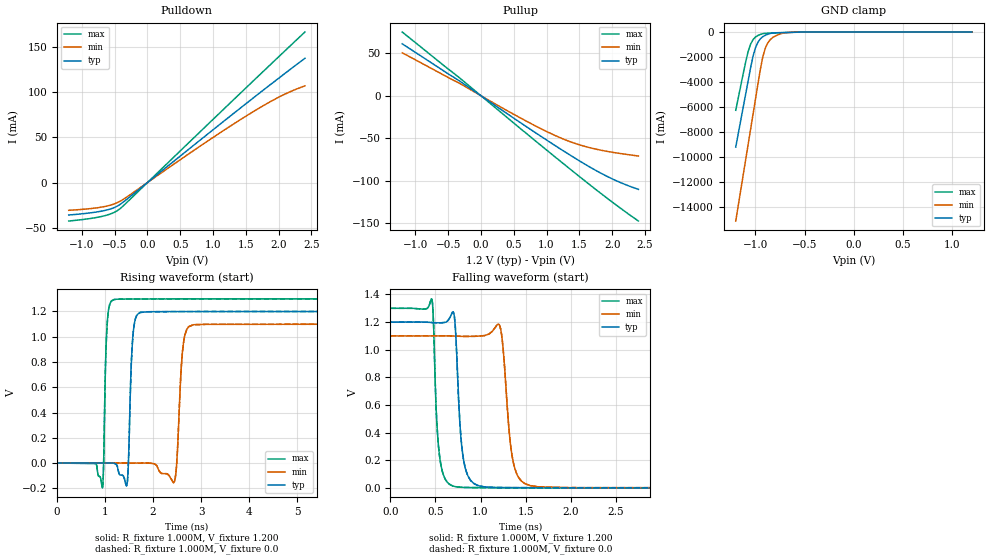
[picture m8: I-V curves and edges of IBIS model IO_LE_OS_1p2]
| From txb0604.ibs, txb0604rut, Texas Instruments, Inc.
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|   Model IO_LE_OS_1p2
[Model] IO_LE_OS_1p2
Model_type 3-state
Polarity   Non-Inverting
Enable   Active-High
Vmeas =  0.600V
Cref =  15.000pF
Rref =  1.000M
Vref =  0.0V
C_comp   3.930pF   3.640pF   4.130pF
[Temperature Range]   27.000   0.125k   -40.000
[Voltage Range]   1.200V   1.100V   1.300V
[Pullup Reference]   1.200V   1.100V   1.300V
[Pulldown Reference]   0.0V   0.0V   0.0V
[POWER Clamp Reference]   1.200V   1.100V   1.300V
[GND Clamp Reference]   0.0V   0.0V   0.0V
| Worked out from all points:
|   slope of the pulldown table from 0 to 0.18 V, typ, clamps not added: 17 ohm
|   slope of the pullup table from 0 to 0.18 V, typ, clamps not added: 18.8 ohm
|   GND clamp passes 1 mA (typ) near -0.43 V on its own axis
|   rising waveform, R_fixture 1.000M, V_fixture 1.200: 20-80 % time 65.4ps typ, 89ps min, 51.2ps max; typ from 0 V to 1.2 V
|   rising waveform, R_fixture 1.000M, V_fixture 0.0: 20-80 % time 65.4ps typ, 89ps min, 51.7ps max; typ from 0 V to 1.2 V
|   falling waveform, R_fixture 1.000M, V_fixture 1.200: 20-80 % time 66.8ps typ, 87ps min, 54.7ps max; typ from 1.2 V to 0 V
|   falling waveform, R_fixture 1.000M, V_fixture 0.0: 20-80 % time 66.8ps typ, 87ps min, 54.7ps max; typ from 1.2 V to 0 V
[Pulldown]
|Voltage   I(typ)   I(min)   I(max)
-1.2V     -35.9mA    -30.68mA   -42.54mA
-682mV    -31.36mA   -26.94mA   -37.24mA
-534mV    -28.49mA   -24.35mA   -33.9mA
-423mV    -24.43mA   -20.91mA   -29.2mA
835mV     48.82mA    41.85mA    58.4mA
1.501V    87.2mA     73.43mA    104.7mA
1.982V    114.4mA    93.71mA    137.9mA
2.204V    126.7mA    101.4mA    153.1mA
2.4V      137.5mA    106.9mA    166.5mA
[Pullup]
|Voltage   I(typ)   I(min)   I(max)
-1.2V     61.16mA    50.59mA    75.06mA
-301mV    16.09mA    13.51mA    19.48mA
624mV     -32.89mA   -27.11mA   -40.09mA
1.179V    -61.14mA   -48.51mA   -75.2mA
1.512V    -77.25mA   -58.08mA   -95.9mA
1.845V    -91.93mA   -64.39mA   -116.1mA
2.141V    -102.8mA   -68.28mA   -133.3mA
2.4V      -110.3mA   -70.97mA   -147.6mA
[GND_clamp]
|Voltage   I(typ)   I(min)   I(max)
-1.2V     -9.186A    -15.09A    -6.25A
-1.075V   -3.941A    -9.027A    -1.583A
-1.025V   -1.957A    -6.601A    -615mA
-1V       -1.272A    -5.388A    -399.7mA
-975mV    -819.4mA   -4.175A    -276mA
-925mV    -369.8mA   -1.974A    -131.5mA
-900mV    -261mA     -1.3A      -105.2mA
-875mV    -181mA     -875mA     -93.58mA
-825mV    -80.65mA   -440mA     -80.5mA
-725mV    -43.5mA    -98.28mA   -56.44mA
-625mV    -20.69mA   -20.96mA   -26.75mA
1.2V      0A         0A         0A
[Ramp]
| variable   typ   min   max
dV/dt_r   0.720/65.666p   0.660/89.357p   0.780/51.468p
dV/dt_f   0.720/66.979p   0.660/87.340p   0.780/54.824p
R_load = 1.000M
[Rising Waveform]
R_fixture= 1.000M
V_fixture= 1.200
V_fixture_min= 1.100
V_fixture_max= 1.300
|time   V(typ)   V(min)   V(max)
0s        20.38uV    23.63uV    18.47uV
950ps     -65.72uV   22.48uV    -190.9mV
1.042ns   -107.5uV   20.14uV    1.083V
1.179ns   -662.1uV   12.7uV     1.294V
1.456ns   -172.9mV   -21.17uV   1.298V
1.581ns   1.01V      -53.87uV   1.299V
1.731ns   1.192V     -58.08uV   1.299V
2.444ns   1.199V     -148mV     1.3V
2.841ns   1.2V       1.095V     1.3V
10ns      1.2V       1.1V       1.3V
[Rising Waveform]
R_fixture= 1.000M
V_fixture= 0.0
V_fixture_min= 0.0
V_fixture_max= 0.0
|time   V(typ)   V(min)   V(max)
0s        -28.04nV   2.03uV     -68.93nV
950ps     -86.16uV   883.5nV    -193.5mV
1.041ns   -127.9uV   -1.421uV   1.075V
1.173ns   -399.4uV   -8.414uV   1.293V
1.456ns   -173mV     -42.8uV    1.298V
1.581ns   1.01V      -75.54uV   1.299V
1.731ns   1.192V     -79.87uV   1.299V
2.444ns   1.199V     -148.1mV   1.3V
2.841ns   1.2V       1.095V     1.3V
10ns      1.2V       1.1V       1.3V
[Falling Waveform]
R_fixture= 1.000M
V_fixture= 1.200
V_fixture_min= 1.100
V_fixture_max= 1.300
|time   V(typ)   V(min)   V(max)
0s        1.2V       1.1V       1.3V
459ps     1.197V     1.1V       1.368V
545ps     1.195V     1.1V       231.1mV
719ps     1.174V     1.099V     9.188mV
801ps     248.4mV    1.097V     3.624mV
981ps     14.38mV    1.099V     1.712mV
1.212ns   2.129mV    1.175V     1.081mV
1.361ns   1.477mV    190.9mV    826uV
1.551ns   1.093mV    16.27mV    632.7uV
10ns      25.52uV    42.77uV    19.7uV
[Falling Waveform]
R_fixture= 1.000M
V_fixture= 0.0
V_fixture_min= 0.0
V_fixture_max= 0.0
|time   V(typ)   V(min)   V(max)
0s        1.2V       1.1V       1.3V
459ps     1.197V     1.1V       1.368V
545ps     1.195V     1.1V       231.1mV
719ps     1.173V     1.099V     9.169mV
801ps     248.3mV    1.097V     3.606mV
981ps     14.36mV    1.099V     1.693mV
1.212ns   2.109mV    1.175V     1.062mV
1.361ns   1.457mV    190.9mV    807.5uV
1.551ns   1.073mV    16.25mV    614.1uV
10ns      5.114uV    21.17uV    1.161uV
